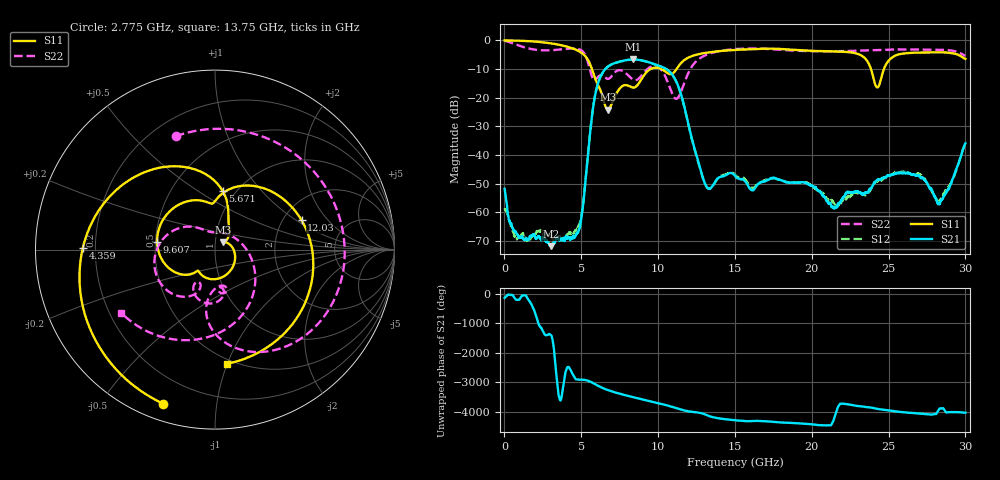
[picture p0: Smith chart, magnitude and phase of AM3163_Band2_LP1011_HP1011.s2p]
!Agilent Technologies,E8364B,MY43040894,A.07.50.67
!Agilent E8364B: A.07.50.67
!Date: Thursday, August 20, 2020 11:14:57
!Correction: S11(Full 2 Port(1,2))
!S21(Full 2 Port(1,2))
!S12(Full 2 Port(1,2))
!S22(Full 2 Port(1,2))
!S2P File: Measurements: S11, S21, S12, S22:
# Hz S  dB  R 50
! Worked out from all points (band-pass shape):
!   3201 points, 10 MHz to 30 GHz, reference 50 ohm
!   highest |S21| = -6.67 dB at 8.398 GHz (marker M1); lowest = -71.8 dB at 3.018 GHz (marker M2)
!   |S21| within 3 dB of the highest: 6.622 GHz to 10.42 GHz (3.802 GHz wide, 44.6 % of centre)
!   lowest |S11| = -24.2 dB at 6.739 GHz (marker M3), VSWR 1.13, Z = 54.7 + j4.42 ohm
!   |S11| at or under -10 dB: 5.692 GHz to 9.509 GHz (3.817 GHz wide, 50.2 % of centre); 10.21 GHz to 11.2 GHz (994.2 MHz wide, 9.29 % of centre); 23.85 GHz to 24.7 GHz (843.4 MHz wide, 3.47 % of centre)
!   |S22| runs from -20.4 to -0.2 dB; largest |S21 - S12| = 0.0037
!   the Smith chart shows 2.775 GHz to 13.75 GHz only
!   S11 on the Smith chart (normalised r, x): 2.775 GHz: 0.08, -0.72; 4.359 GHz: 0.15, +0.01; 5.671 GHz: 0.87, +0.64; 9.607 GHz: 0.51, +0.05; 12.03 GHz: 2.51, +1.11; 13.75 GHz: 0.46, -1.00
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1e7  -0.04 -2.9  -51.79 -134.5  -58.55 -15.8  -0.18 -8.4
6.941469e8  -0.08 -26.6  -66.86 -161.8  -68.63 -61.8  -1.34 -79.1
1.462641e9  -0.23 -56.4  -69.23 -116.9  -69.68 -64.4  -2.68 -151.1
2.774703e9  -0.86 -108.6  -70.38 39.9  -67.98 150.0  -3.50 109.1
3.018372e9  -1.04 -118.7  -71.78 40.0  -68.57 -75.7  -3.45 92.2
4.35855e9  -2.66 179.1  -68.70 -128.6  -67.24 -140.6  -2.82 -0.1
5.014581e9  -4.35 138.5  -61.68 -35.5  -60.86 -36.1  -3.51 -54.2
5.670612e9  -9.67 82.4  -27.53 -125.2  -27.56 -125.4  -12.26 -95.1
6.739006e9  -24.20 40.7  -9.13 -31.3  -9.15 -31.5  -13.44 -82.0
7.648078e9  -16.05 -73.0  -7.20 -175.4  -7.25 -175.3  -10.55 -105.6
8.397828e9  -16.47 -128.5  -6.67 84.9  -6.69 85.0  -13.73 -118.9
9.6068e9  -9.76 172.8  -8.01 -65.0  -8.04 -65.2  -9.05 -141.6
1.000979e10  -9.62 139.8  -8.75 -114.2  -8.80 -114.3  -9.37 -171.5
1.203412e10  -5.86 18.7  -30.69 -37.6  -30.91 -37.5  -10.67 -40.2
1.374917e10  -3.88 -83.9  -48.98 107.5  -49.16 108.0  -4.01 -146.2
1.5005e10  -3.33 -138.2  -47.21 19.0  -46.87 21.4  -3.05 162.9
1.779782e10  -2.96 96.5  -48.42 -45.8  -48.47 -48.0  -3.24 49.7
2.000958e10  -3.67 -16.2  -50.68 -115.1  -51.04 -122.2  -3.79 -35.8
2.302732e10  -4.79 -140.3  -52.83 145.8  -53.17 143.3  -3.60 -125.7
2.500479e10  -7.08 -131.2  -47.22 -7.0  -47.51 -3.5  -3.29 -174.7
2.831306e10  -4.17 110.5  -57.08 55.8  -56.00 90.5  -3.26 99.0
3e10  -6.47 47.7  -35.90 -81.9  -36.26 -80.1  -5.41 48.6
